| TEXAS INSTRUMENTS INCORPORATED
| Standard Linear and Logic Group
| IBIS Model of SN74ALVCH162260
| 12-BIT TO 24-BIT MULTIPLEXED D-TYPE LATCH WITH 3-STATE OUTPUTS
| This file contains package information for the following:
|  TSSOP 56-pin (DGG) package as [Component] ALVCH162260_DGG
|  SSOP 56-pin (DL) package as [Component] ALVCH162260_DL
| This device can be powered at the following Vccs:
|  1.8 volt Vcc
|  2.5 volt Vcc
|  2.7 volt Vcc
|  3.3 volt Vcc
| This file provides unique models under the [Model Selector] for each Vcc.
| For operation at a specific Vcc, select the appropriate model after each
| [Model Selector] keyword.
[IBIS Ver]   3.2
[Comment char]  |_char
[File Name]   sn74alvch162260.ibs
[File Rev]   1.1 | b_die
[Date]   April 10, 2003
[Source]   Data created from TI-SPICE simulations at TI-SLL.
[Notes]   The following is an IBIS list for the SN74ALVCH162260.
   Please contact sllibis@ti.com with questions and
   comments concerning SLL IBIS models.
   This IBIS model is created from a BA (back annotated
   netlist).
   - C_comp values are taken at a different test condition than
   the Ci in data sheet.
   - Due to presence of bus hold at input, GND-clamp curves
   have non-monotonic warnings.
   - Non-monotonic data in pullup data due to resistor at output.
[Disclaimer] Property of Texas Instruments Incorporated. Unauthorized
   reproduction and/or distribution is strictly prohibited.
   This product is protected under copyright law.
   Created 2003,(C) Copyright 2003, Texas Instruments
   Incorporated, All Rights Reserved
   UNLESS THERE IS A SIGNED, WRITTEN AGREEMENT TO THE
   CONTRARY, TEXAS INSTRUMENTS (TI) IS PROVIDING THE IBIS
   MODELS AND WITHOUT ANY WARRANTY, EXPRESSED OR
   IMPLIED. TI assumes no liability for:
   1) the accuracy of the IBIS models provided to your
   company;
   2) the proper functioning of these IBIS Models in your
   design or for any resulting applications; or
   3) infringement of patents, copyrights or intellectual
   property rights resulting from your use of these IBIS
   models.
   TI provides IBIS Models as a service to our customers.
   You and your company shall not distribute, sell or give
   these models to anyone else without prior written
   permission from TI.
   TI reserves the right to make changes to our products or
   to discontinue any semiconductor product or service
   without notice, and advises our customers to obtain the
   latest version of relevant information to verify, before
   placing orders, that the information being relied on is
   current.
   Please be aware that your receipt and use of the IBIS
   information provided shall serve as acceptance of these
   terms and conditions. If you do not accept these terms,
   you should return or destroy the IBIS models and any
   other accompanying information immediately.
| Component ALVCH162260_DGG 56-pin TSSOP
[Component]   ALVCH162260_DGG
[Manufacturer]   Texas Instruments, Inc.
[Package]
|   typ   min   max
R_pkg   4.500e-02   3.500e-02   6.200e-02
L_pkg   3.324e-09   2.403e-09   5.094e-09
C_pkg   5.640e-13   3.410e-13   9.140e-13
[Pin]   signal_name   model_name   R_pin   L_pin   C_pin
1   NOEA   ALVCH162260_OEA   6.200e-02   5.094e-09   8.560e-13
2   LE1B   ALVCH162260_LEB   6.100e-02   4.621e-09   9.020e-13
3   2B3   ALVCH162260_BIO   6.000e-02   4.316e-09   8.020e-13
4   GND   GND   5.900e-02   3.968e-09   6.980e-13
5   2B2   ALVCH162260_BIO   5.700e-02   3.716e-09   6.490e-13
6   2B1   ALVCH162260_BIO   4.200e-02   3.517e-09   6.530e-13
7   VCC   POWER   4.100e-02   3.160e-09   5.700e-13
8   A1   ALVCH162260_AIO   3.900e-02   2.981e-09   4.820e-13
9   A2   ALVCH162260_AIO   3.900e-02   2.808e-09   4.470e-13
10   A3   ALVCH162260_AIO   3.800e-02   2.715e-09   4.090e-13
11   GND   GND   4.100e-02   2.675e-09   3.910e-13
12   A4   ALVCH162260_AIO   3.900e-02   2.536e-09   3.660e-13
13   A5   ALVCH162260_AIO   3.900e-02   2.457e-09   3.480e-13
14   A6   ALVCH162260_AIO   3.800e-02   2.411e-09   3.530e-13
15   A7   ALVCH162260_AIO   3.900e-02   2.456e-09   3.550e-13
16   A8   ALVCH162260_AIO   3.900e-02   2.471e-09   3.490e-13
17   A9   ALVCH162260_AIO   4.000e-02   2.580e-09   3.700e-13
18   GND   GND   3.800e-02   2.651e-09   3.890e-13
19   A10   ALVCH162260_AIO   3.800e-02   2.739e-09   4.110e-13
20   A11   ALVCH162260_AIO   3.900e-02   2.838e-09   4.490e-13
21   A12   ALVCH162260_AIO   3.800e-02   2.988e-09   4.840e-13
22   VCC   POWER   3.800e-02   3.104e-09   5.640e-13
23   1B1   ALVCH162260_BIO   4.000e-02   3.427e-09   6.380e-13
24   1B2   ALVCH162260_BIO   5.600e-02   3.654e-09   6.410e-13
25   GND   GND   5.700e-02   3.932e-09   7.000e-13
26   1B3   ALVCH162260_BIO   5.800e-02   4.257e-09   8.060e-13
27   LE2B   ALVCH162260_LEB   5.700e-02   4.580e-09   9.140e-13
28   SEL   ALVCH162260_SEL   5.900e-02   5.038e-09   8.610e-13
29   NOE1B   ALVCH162260_OEB   6.000e-02   5.058e-09   8.580e-13
30   LEA1B   ALVCH162260_LEAB   5.600e-02   4.543e-09   9.040e-13
31   1B4   ALVCH162260_BIO   5.700e-02   4.241e-09   8.020e-13
32   GND   GND   5.900e-02   3.933e-09   6.990e-13
33   1B5   ALVCH162260_BIO   5.600e-02   3.616e-09   6.370e-13
34   1B6   ALVCH162260_BIO   3.700e-02   3.368e-09   6.400e-13
35   VCC   POWER   3.600e-02   3.024e-09   5.630e-13
36   1B7   ALVCH162260_BIO   3.500e-02   2.876e-09   4.740e-13
37   1B8   ALVCH162260_BIO   3.500e-02   2.745e-09   4.440e-13
38   1B9   ALVCH162260_BIO   3.700e-02   2.683e-09   4.050e-13
39   GND   GND   3.800e-02   2.603e-09   3.820e-13
40   1B10   ALVCH162260_BIO   3.800e-02   2.510e-09   3.620e-13
41   1B11   ALVCH162260_BIO   3.600e-02   2.412e-09   3.410e-13
42   1B12   ALVCH162260_BIO   3.800e-02   2.416e-09   3.490e-13
43   2B12   ALVCH162260_BIO   3.800e-02   2.403e-09   3.490e-13
44   2B11   ALVCH162260_BIO   3.700e-02   2.429e-09   3.410e-13
45   2B10   ALVCH162260_BIO   3.600e-02   2.483e-09   3.580e-13
46   GND   GND   3.700e-02   2.614e-09   3.810e-13
47   2B9   ALVCH162260_BIO   3.500e-02   2.669e-09   4.020e-13
48   2B8   ALVCH162260_BIO   3.600e-02   2.763e-09   4.420e-13
49   2B7   ALVCH162260_BIO   3.600e-02   2.942e-09   4.780e-13
50   VCC   POWER   3.500e-02   3.053e-09   5.640e-13
51   2B6   ALVCH162260_BIO   3.600e-02   3.408e-09   6.410e-13
52   2B5   ALVCH162260_BIO   5.800e-02   3.698e-09   6.410e-13
53   GND   GND   5.900e-02   3.974e-09   6.970e-13
54   2B4   ALVCH162260_BIO   6.100e-02   4.327e-09   8.020e-13
55   LEA2B   ALVCH162260_LEAB   6.100e-02   4.624e-09   9.050e-13
56   NOE2B   ALVCH162260_OEB   6.000e-02   5.063e-09   8.580e-13
| Component ALVCH162260_DL 56-pin SSOP
[Component]   ALVCH162260_DL
[Manufacturer]   Texas Instruments, Inc.
[Package]
|   typ   min   max
R_pkg   5.500e-02   4.800e-02   6.700e-02
L_pkg   6.539e-09   4.803e-09   9.746e-09
C_pkg   8.570e-13   5.000e-13   1.351e-12
[Pin]   signal_name   model_name   R_pin   L_pin   C_pin
1   NOEA   ALVCH162260_OEA   6.400e-02   9.646e-09   1.202e-12
2   LE1B   ALVCH162260_LEB   5.900e-02   8.723e-09   1.348e-12
3   2B3   ALVCH162260_BIO   5.900e-02   8.139e-09   1.223e-12
4   GND   GND   5.600e-02   7.554e-09   1.088e-12
5   2B2   ALVCH162260_BIO   5.400e-02   6.991e-09   9.660e-13
6   2B1   ALVCH162260_BIO   5.300e-02   6.659e-09   9.730e-13
7   VCC   POWER   5.500e-02   6.321e-09   9.050e-13
8   A1   ALVCH162260_AIO   5.600e-02   5.942e-09   7.130e-13
9   A2   ALVCH162260_AIO   5.700e-02   5.768e-09   6.780e-13
10   A3   ALVCH162260_AIO   5.400e-02   5.459e-09   6.310e-13
11   GND   GND   5.100e-02   5.224e-09   6.380e-13
12   A4   ALVCH162260_AIO   4.800e-02   5.088e-09   6.010e-13
13   A5   ALVCH162260_AIO   5.000e-02   5.021e-09   5.180e-13
14   A6   ALVCH162260_AIO   5.100e-02   4.803e-09   5.000e-13
15   A7   ALVCH162260_AIO   5.100e-02   4.803e-09   5.000e-13
16   A8   ALVCH162260_AIO   5.000e-02   5.021e-09   5.180e-13
17   A9   ALVCH162260_AIO   4.800e-02   5.088e-09   6.010e-13
18   GND   GND   5.100e-02   5.224e-09   6.380e-13
19   A10   ALVCH162260_AIO   5.400e-02   5.459e-09   6.310e-13
20   A11   ALVCH162260_AIO   5.700e-02   5.768e-09   6.770e-13
21   A12   ALVCH162260_AIO   5.500e-02   5.942e-09   7.150e-13
22   VCC   POWER   5.500e-02   6.321e-09   9.070e-13
23   1B1   ALVCH162260_BIO   5.300e-02   6.659e-09   9.720e-13
24   1B2   ALVCH162260_BIO   5.400e-02   6.991e-09   9.660e-13
25   GND   GND   5.600e-02   7.554e-09   1.087e-12
26   1B3   ALVCH162260_BIO   5.900e-02   8.139e-09   1.223e-12
27   LE2B   ALVCH162260_LEB   5.900e-02   8.727e-09   1.351e-12
28   SEL   ALVCH162260_SEL   6.700e-02   9.746e-09   1.210e-12
29   NOE1B   ALVCH162260_OEB   6.300e-02   9.630e-09   1.203e-12
30   LEA1B   ALVCH162260_LEAB   6.000e-02   8.751e-09   1.349e-12
31   1B4   ALVCH162260_BIO   6.000e-02   8.184e-09   1.224e-12
32   GND   GND   5.600e-02   7.543e-09   1.087e-12
33   1B5   ALVCH162260_BIO   5.400e-02   7.005e-09   9.690e-13
34   1B6   ALVCH162260_BIO   5.600e-02   6.714e-09   9.750e-13
35   VCC   POWER   5.800e-02   6.384e-09   9.090e-13
36   1B7   ALVCH162260_BIO   5.700e-02   5.976e-09   7.170e-13
37   1B8   ALVCH162260_BIO   5.700e-02   5.743e-09   6.770e-13
38   1B9   ALVCH162260_BIO   5.400e-02   5.468e-09   6.310e-13
39   GND   GND   5.500e-02   5.329e-09   6.440e-13
40   1B10   ALVCH162260_BIO   5.200e-02   5.189e-09   6.060e-13
41   1B11   ALVCH162260_BIO   5.200e-02   5.053e-09   5.190e-13
42   1B12   ALVCH162260_BIO   5.200e-02   4.825e-09   5.020e-13
43   2B12   ALVCH162260_BIO   5.400e-02   4.897e-09   5.060e-13
44   2B11   ALVCH162260_BIO   5.200e-02   5.093e-09   5.210e-13
45   2B10   ALVCH162260_BIO   5.100e-02   5.179e-09   6.080e-13
46   GND   GND   5.400e-02   5.314e-09   6.450e-13
47   2B9   ALVCH162260_BIO   5.500e-02   5.511e-09   6.320e-13
48   2B8   ALVCH162260_BIO   5.700e-02   5.770e-09   6.770e-13
49   2B7   ALVCH162260_BIO   5.600e-02   5.956e-09   7.160e-13
50   VCC   POWER   5.500e-02   6.320e-09   9.050e-13
51   2B6   ALVCH162260_BIO   5.200e-02   6.621e-09   9.680e-13
52   2B5   ALVCH162260_BIO   5.300e-02   6.974e-09   9.660e-13
53   GND   GND   5.700e-02   7.571e-09   1.089e-12
54   2B4   ALVCH162260_BIO   5.700e-02   8.097e-09   1.219e-12
55   LEA2B   ALVCH162260_LEAB   5.900e-02   8.723e-09   1.349e-12
56   NOE2B   ALVCH162260_OEB   6.100e-02   9.560e-09   1.199e-12
| Model ALVCH162260_LEAB
[Model Selector]   ALVCH162260_LEAB
ALVCH162260_LEAB_18   1.8 volt Vcc
ALVCH162260_LEAB_25   2.5 volt Vcc
ALVCH162260_LEAB_27   2.7 volt Vcc
ALVCH162260_LEAB_33   3.3 volt Vcc
| Model ALVCH162260_SEL
[Model Selector]   ALVCH162260_SEL
ALVCH162260_SEL_18   1.8 volt Vcc
ALVCH162260_SEL_25   2.5 volt Vcc
ALVCH162260_SEL_27   2.7 volt Vcc
ALVCH162260_SEL_33   3.3 volt Vcc
| Model ALVCH162260_LEB
[Model Selector]   ALVCH162260_LEB
ALVCH162260_LEB_18   1.8 volt Vcc
ALVCH162260_LEB_25   2.5 volt Vcc
ALVCH162260_LEB_27   2.7 volt Vcc
ALVCH162260_LEB_33   3.3 volt Vcc
| Model ALVCH162260_OEA
[Model Selector]   ALVCH162260_OEA
ALVCH162260_OEA_18   1.8 volt Vcc
ALVCH162260_OEA_25   2.5 volt Vcc
ALVCH162260_OEA_27   2.7 volt Vcc
ALVCH162260_OEA_33   3.3 volt Vcc
| Model ALVCH162260_OEB
[Model Selector]   ALVCH162260_OEB
ALVCH162260_OEB_18   1.8 volt Vcc
ALVCH162260_OEB_25   2.5 volt Vcc
ALVCH162260_OEB_27   2.7 volt Vcc
ALVCH162260_OEB_33   3.3 volt Vcc
| Model ALVCH162260_AIO
[Model Selector]   ALVCH162260_AIO
ALVCH162260_AIO_18   1.8 volt Vcc
ALVCH162260_AIO_25   2.5 volt Vcc
ALVCH162260_AIO_27   2.7 volt Vcc
ALVCH162260_AIO_33   3.3 volt Vcc
| Model ALVCH162260_BIO
[Model Selector]   ALVCH162260_BIO
ALVCH162260_BIO_18   1.8 volt Vcc
ALVCH162260_BIO_25   2.5 volt Vcc
ALVCH162260_BIO_27   2.7 volt Vcc
ALVCH162260_BIO_33   3.3 volt Vcc
| Models and submodels in the file (28): ALVCH162260_LEAB_18 (Input), ALVCH162260_LEAB_25 (Input), ALVCH162260_LEAB_27 (Input), ALVCH162260_LEAB_33 (Input), ALVCH162260_SEL_18 (Input), ALVCH162260_SEL_25 (Input), ALVCH162260_SEL_27 (Input), ALVCH162260_SEL_33 (Input), ALVCH162260_LEB_18 (Input), ALVCH162260_LEB_25 (Input), ALVCH162260_LEB_27 (Input), ALVCH162260_LEB_33 (Input), ALVCH162260_OEA_18 (Input), ALVCH162260_OEA_25 (Input), ALVCH162260_OEA_27 (Input), ALVCH162260_OEA_33 (Input), ALVCH162260_OEB_18 (Input), ALVCH162260_OEB_25 (Input), ALVCH162260_OEB_27 (Input), ALVCH162260_OEB_33 (Input), ALVCH162260_AIO_18 (I/O), ALVCH162260_AIO_25 (I/O), ALVCH162260_AIO_27 (I/O), ALVCH162260_AIO_33 (I/O), ALVCH162260_BIO_18 (I/O), ALVCH162260_BIO_25 (I/O), ALVCH162260_BIO_27 (I/O), ALVCH162260_BIO_33 (I/O)
